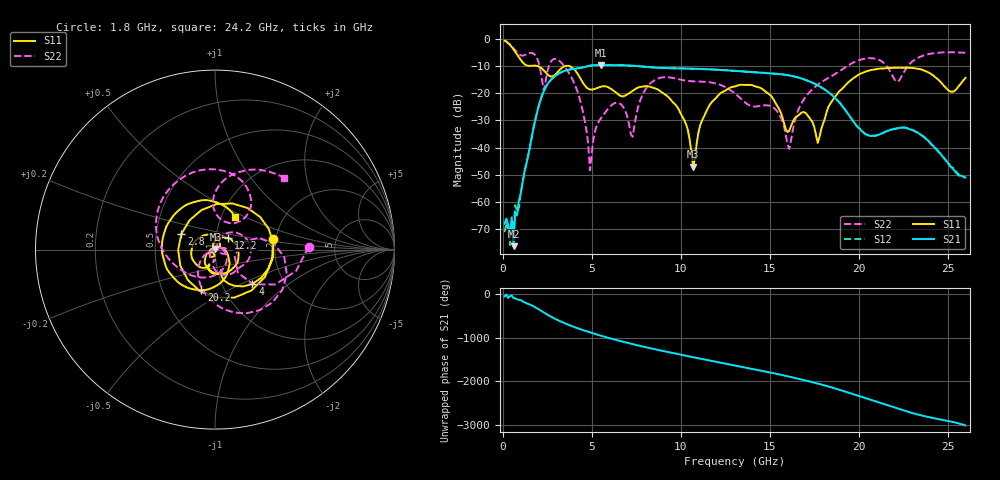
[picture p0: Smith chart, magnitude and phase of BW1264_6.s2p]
!Keysight Technologies,N5245B,MY57181159,A.13.60.06
!Date: Friday, December 18, 2020 23:52:13
!Correction: S11(Full 2 Port(1,2))
!S21(Full 2 Port(1,2))
!S12(Full 2 Port(1,2))
!S22(Full 2 Port(1,2))
!S2P File: Measurements: S11, S21, S12, S22:
# Hz S  dB  R 50
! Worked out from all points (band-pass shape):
!   260 points, 100 MHz to 26 GHz, reference 50 ohm
!   highest |S21| = -9.46 dB at 5.5 GHz (marker M1); lowest = -76.5 dB at 600 MHz (marker M2)
!   |S21| within 3 dB of the highest: 3.188 GHz to 14.78 GHz (11.59 GHz wide, 129 % of centre)
!   lowest |S11| = -47.1 dB at 10.7 GHz (marker M3), VSWR 1.01, Z = 50.2 + j0.379 ohm
!   |S11| at or under -10 dB: 2.01 GHz to 3.455 GHz (1.445 GHz wide, 52.9 % of centre); 3.791 GHz to end of sweep
!   |S22| runs from -48.4 to -0.4 dB; largest |S21 - S12| = 0.00057
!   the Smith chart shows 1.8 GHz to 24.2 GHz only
!   S11 on the Smith chart (normalised r, x): 1.8 GHz: 1.93, +0.26; 2.8 GHz: 0.68, +0.12; 4 GHz: 1.39, -0.58; 12.2 GHz: 1.15, +0.15; 20.2 GHz: 0.78, -0.37; 24.2 GHz: 1.16, +0.44
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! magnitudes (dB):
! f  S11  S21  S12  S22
! 100 MHz  -0.5  -68.2  -71.3  -0.4
! 600 MHz  -3.7  -76.5  -69.1  -3.2
! 1.8 GHz  -9.7  -30.5  -30.5  -5.7
! 2.3 GHz  -11.4  -19.1  -19.1  -18.8
! 2.8 GHz  -13.7  -14.3  -14.3  -7.5
! 4 GHz  -11.0  -10.9  -10.9  -15.9
! 4.5 GHz  -16.0  -10.4  -10.3  -26.7
! 4.9 GHz  -18.5  -9.7  -9.7  -48.4
! 5.5 GHz  -17.5  -9.5  -9.5  -29.3
! 7.3 GHz  -19.0  -9.7  -9.7  -36.0
! 8.8 GHz  -18.9  -10.5  -10.5  -14.3
! 10.3 GHz  -31.4  -10.8  -10.8  -15.3
! 10.7 GHz  -47.1  -10.8  -10.8  -15.5
! 12.2 GHz  -20.1  -11.3  -11.3  -16.8
! 13.1 GHz  -17.3  -11.7  -11.7  -20.3
! 16.1 GHz  -33.8  -13.3  -13.3  -40.5
! 17.4 GHz  -30.5  -16.0  -16.0  -18.4
! 17.7 GHz  -38.3  -17.0  -17.0  -16.8
! 20.2 GHz  -12.4  -34.1  -34.1  -7.3
! 21.7 GHz  -10.6  -33.7  -33.6  -11.0
! 24.2 GHz  -13.4  -39.4  -39.4  -5.1
! 26 GHz  -14.2  -51.1  -51.1  -5.0
